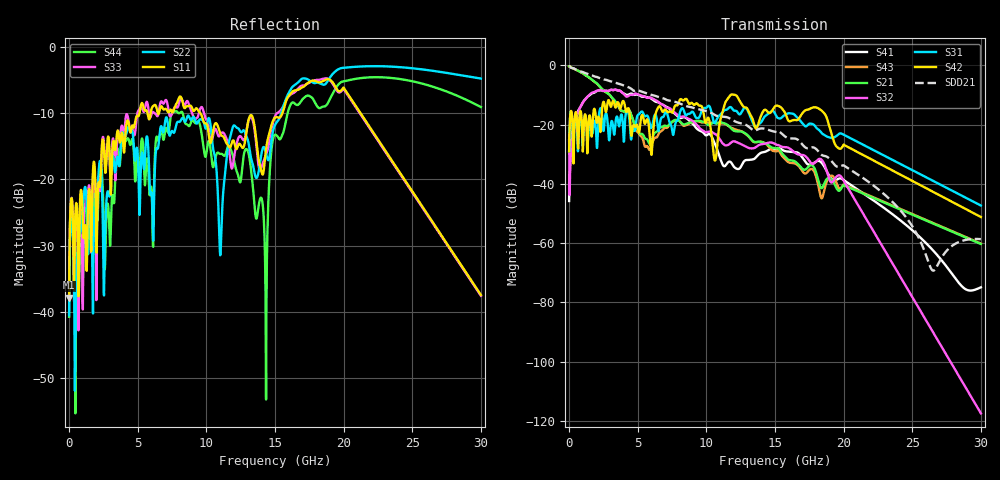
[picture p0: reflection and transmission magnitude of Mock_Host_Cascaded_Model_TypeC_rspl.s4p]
# Hz S RI R 50
! S-Parameters data
! Freq  reS11  imS11  reS12  imS12  reS13  imS13  reS14  imS14
!  reS21  imS21  reS22  imS22  reS23  imS23  reS24  imS24
!  reS31  imS31  reS32  imS32  reS33  imS33  reS34  imS34
!  reS41  imS41  reS42  imS42  reS43  imS43  reS44  imS44
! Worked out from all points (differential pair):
!   1500 points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, 20 MHz to 30 GHz, reference 50 ohm
!   strongest paths, dB at 20 MHz, 7.52 GHz, 15.02 GHz, 22.52 GHz, 30 GHz:
!     S42: -29.1, -16.0, -13.8, -32.9, -51.2
!     S31: -29.0, -21.8, -16.4, -29.4, -47.3
!     S32: -25.2, -15.1, -26.6, -58.7, -117.5
!     S21: -0.4, -19.0, -28.0, -45.5, -60.3
!     S43: -0.4, -19.2, -29.0, -45.2, -60.1
!     S41: -45.8, -15.6, -28.4, -46.7, -74.9
!   taken as a pair (ports 1,3 in; 2,4 out), SDD21 dB: -0.4, -12.1, -22.4, -41.8, -58.7
!   lowest |S11| = -37.8 dB at 20 MHz (marker M1), VSWR 1.03, Z = 50.9 - j0.895 ohm
!   |S11| at or under -10 dB: start of sweep to 5.144 GHz; 9.576 GHz to 15.55 GHz (5.977 GHz wide, 47.6 % of centre); 21.23 GHz to end of sweep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
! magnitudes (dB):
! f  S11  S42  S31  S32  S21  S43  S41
! 20 MHz  -37.8  -29.1  -29.0  -25.2  -0.4  -0.4  -45.8
! 1.28 GHz  -33.0  -20.5  -19.6  -11.0  -3.5  -3.5  -11.0
! 5.78 GHz  -10.6  -19.2  -17.5  -10.9  -25.8  -27.8  -10.8
! 14.34 GHz  -15.7  -15.1  -17.0  -26.4  -26.4  -26.5  -29.1
! 18.02 GHz  -5.2  -14.2  -21.1  -32.4  -36.5  -37.9  -32.4
! 25.24 GHz  -22.5  -39.6  -35.9  -80.0  -50.9  -50.7  -56.6
! 30 GHz  -37.4  -51.2  -47.3  -117.5  -60.3  -60.1  -74.9
